| IBIS file stm32mp157xac_tfbga361.ibs
[IBIS ver]   4.2
[File name]   stm32mp157xac_tfbga361.ibs
[File Rev]   2.2
[Date]   07-07-2026
[Source]   Data Created at STMicroelectronics
[Disclaimer]  This information is for modeling purpose only and is
   not guaranted.
   The information is subject to change without notice.
[Copyright]   Copyright 2026 STMicroelectronics Inc.
|   Component stm32mp157xac_tfbga361
[Component] stm32mp157xac_tfbga361
[Manufacturer] STMicroelectronics
[Package]
| variable   typ   min   max
R_pkg  4.84E-01  2.14E-01  8.53E-01
L_pkg  2.71E-09  1.27E-09  5.07E-09
C_pkg  7.70E-13  5.20E-13  3.84E-12
[Pin]   signal_name   model_name
1A2  VDDCORE  power
1A3  VSS  gnd
1A4  VDDCORE  power
1A5  VSS  gnd
1A6  VDDCORE  power
1A7  VSS  gnd
1A8  VDDQ_DDR  power
1B1  VDDCORE  power
1B2  VSS  gnd
1B3  VDDCORE  power
1B4  VSS  gnd
1B5  VDDCORE  power
1B6  VSS  gnd
1B7  VDDQ_DDR  power
1B8  VSS  gnd
1B9  VDDQ_DDR  power
1C1  VSS  gnd
1C2  VDDCORE  power
1C3  VSS  gnd
1C4  VDDCORE  power
1C5  VSS  gnd
1C6  VDDCORE  power
1C7  VSS  gnd
1C8  VDDQ_DDR  power
1C9  VSS  gnd
1D1  VDDCORE  power
1D2  VSS  gnd
1D3  VDDCORE  power
1D4  VSS  gnd
1D5  VDDCORE  power
1D6  VSS  gnd
1D7  VDDCORE  power
1D8  VSS  gnd
1D9  VDDQ_DDR  power
1E1  VSS  gnd
1E2  VDDCORE  power
1E3  VSS  gnd
1E4  VDDCORE  power
1E5  VSS  gnd
1E6  VDDCORE  power
1E7  VSS  gnd
1E8  VDDQ_DDR  power
1E9  VSS  gnd
1F1  VBAT  power
1F2  VSS  gnd
1F3  VDD  power
1F4  VSS  gnd
1F5  VDDCORE  power
1F6  VSS  gnd
1F7  VDDCORE  power
1F8  VSS  gnd
1F9  VDDQ_DDR  power
1G1  VSS_ANA  nc
1G2  VDD_ANA  nc
1G3  VSS  gnd
1G4  VDD  power
1G5  VSS  gnd
1G6  VDDCORE  power
1G7  VSS  gnd
1G8  VDDQ_DDR  power
1G9  VSS  gnd
1H1  VDDA  nc
1H2  VSSA  gnd
1H3  VDD  power
1H4  VSS  gnd
1H5  VDD  power
1H6  VSS  gnd
1H7  VDDCORE  power
1H8  VSS  gnd
1H9  VDDQ_DDR  power
1J2  VDD_OTP  power
1J3  VSS  gnd
1J4  VDD  power
1J5  VSS  gnd
1J6  VDD  power
1J7  VSS  gnd
1J8  VDDQ_DDR  power
A1  VSS  gnd
A2  PH5  io8_ft_i2c
A3  PE13  io8_ft_hslv
A4  PE11  io8_ft
A5  PF1  io8_ft_hslv
A7  PD5  io8_ft_hslv
A8  PA9  io8_ft_hslv
A10  PG6  io8_ft_hslv
A11  PB3  io8_ft_hslv
A13  PA8  io8_ft_hslv
A14  PF2  io8_ft_hslv
A16  DNU  nc
A17  DNU  nc
A19  JTDO-TRACESWO io8_ft_hslv
A20  JTDI  isudqf
A21  DDR_DQ20  PDDRIO_PAD
A22  DDR_DQ23  PDDRIO_PAD
A23  VSS  gnd
AA1  PG14  io8_ft_hslv_et
AA2  PG13  io8_ft_hslv_et
AA3  PH3  io8_ft_hslv
AA4  PA1  io8_ft_hslv
AA5  VSS  gnd
AA6  PC1  io8_ft_hslv
AA7  PB1  io8_ft
AA8  VSS  gnd
AA9  PE9  io8_ft_hslv
AA10  PB13  io8_ft_hslv_et
AA11  PE7  io8_ft_hslv
AA12  VSS  gnd
AA13  PF6  io8_ft_hslv
AA14  PF9  io8_ft_hslv
AA15  VDD3V3_USBHS  power
AA16  VSS_USBHS  gnd
AA17  VDD3V3_USBFS  power
AA18  PA11  io8_i2c_usb_lsfs_bcd_otg20_ft
AA19  PD13  io8_ft_i2c_hslv
AA20  DDR_DQM3  PDDRIO_PAD
AA21  VSS  gnd
AA22  DDR_DQ31  PDDRIO_PAD
AA23  DDR_DQ30  PDDRIO_PAD
AB1  PB11  io8_ft_et_i2c_hslv
AB2  PG4  io8_ft_hslv_et
AB3  PA0  io8_ft_hslv
AB4  PH2  io8_ft_hslv
AB5  PC0  io8_ft_hslv
AB6  PB0  io8_ft
AB7  PC5  io8_ft
AB8  PA7  io8_ft_hslv
AB9  PG8  io8_ft_hslv_et
AB10  PB8  io8_ft_et_i2c_hslv
AB11  PG10  io8_ft_hslv
AB12  PF7  io8_ft_hslv
AB13  BYPASS_REG1V8  isudqf
AB14  VDDA1V8_REG  nc
AB15  VDDA1V1_REG  nc
AB16  USB_DM2  nc
AB17  USB_DM1  nc
AB18  USB_RREF  nc
AB19  PA12  io8_i2c_usb_lsfs_bcd_otg20_ft
AB20  DDR_DQ27  PDDRIO_PAD
AB21  DDR_DQ26  PDDRIO_PAD
AB22  DDR_DQS3P  PDIFF_PAD
AB23  DDR_DQS3N  PDIFF_PAD
AC1  VSS  gnd
AC2  PG0  io8_ft_hslv_et
AC3  PA2  io8_ft_hslv
AC4  PF14  io8_ft_i2c_hslv
AC5  PB12  io8_ft_hslv_et
AC7  PC4  io8_ft
AC8  PA6  io8_ft_hslv
AC10  PD11  io8_ft_hslv
AC11  PF8  io8_ft_hslv
AC13  PE8  io8_ft_hslv
AC14  PG7  io8_ft_hslv
AC16  USB_DP2  nc
AC17  USB_DP1  nc
AC19  OTG_VBUS  io8usb_vbus_otg20_ft
AC20  DDR_VREF  POWER
AC21  DDR_DQ29  PDDRIO_PAD
AC22  DDR_DQ28  PDDRIO_PAD
AC23  VSS  gnd
B1  PH15  io8_ft
B2  PH12  io8_ft_i2c
B3  PH4  io8_ft_i2c
B4  PE12  io8_ft_hslv
B5  PD10  io8_ft_hslv
B6  PD4  io8_ft_hslv
B7  PG15  io8_ft_hslv
B8  PD0  io8_ft_hslv
B9  PD1  io8_ft_hslv
B10  PB9  io8_ft_hslv
B11  PC7  io8_ft_hslv
B12  PB15  io8_ft_hslv
B13  PB4  io8_ft_hslv
B14  PC6  io8_ft_hslv
B15  DNU  nc
B16  DNU  nc
B17  DNU  nc
B18  VDD_Unused  power
B19  NJTRST  isudqf
B20  JTCK-SWCLK  io8_ft
B21  DDR_DQ19  PDDRIO_PAD
B22  DDR_DQ16  PDDRIO_PAD
B23  DDR_DQS2N  PDIFF_PAD
C1  PI0  io8_ft
C2  PH10  io8_ft
C3  PH14  io8_ft
C4  PH11  io8_ft_i2c
C5  PH9  io8_ft
C6  PE14  io8_ft_hslv
C7  VSS  gnd
C8  PE1  io8_ft
C9  PE3  io8_ft_hslv
C10  PE6  io8_ft_hslv
C11  PE5  io8_ft_hslv
C12  VSS  gnd
C13  PB14  io8_ft_hslv
C14  VDDA1V8_Unused  nc
C15  DNU  nc
C16  VSS  gnd
C17  VDD1V2_Unused   nc
C18  VDD1V2_Unused   nc
C19  PA15  io8_ft_hslv
C20  JTMS-SWDIO  io8_ft_hslv
C21  VSS  gnd
C22  DDR_DQS2P  PDIFF_PAD
C23  DDR_DQM2 PDDRIO_PAD
D1  PH13  io8_ft
D2  PD6  io8_ft_hslv
D3  PE15  io8_ft
D4  VSS  gnd
D5  PH8  io8_ft_i2c
D6  PE0  io8_ft_hslv
D7  PF5  io8_ft_hslv
D8  PF0  io8_ft_hslv
D9  PF4  io8_ft_hslv
D10  PD7  io8_ft_hslv
D11  PB7  io8_ft_hslv
D12  PD2  io8_ft_hslv
D13  PC12  io8_ft_hslv
D14  PD3  io8_ft_hslv
D15  PC10  io8_ft_hslv
D16  PC11  io8_ft_hslv
D17  PC9  io8_ft_hslv
D18  PC8  io8_ft_hslv
D19  PE4  io8_ft_hslv
D20  DDR_RESETN  PDDRIO_PAD
D21  DDR_DQ22  PDDRIO_PAD
D22  DDR_DQ17  PDDRIO_PAD
D23  DDR_DQ18  PDDRIO_PAD
E1  PI3  io8_ft_hslv
E2  PI2  io8_ft_hslv
E3  PI1  io8_ft_hslv
E4  PI4  io8_ft
E20  DDR_A7  PDDRIO_PAD
E21  DDR_DQ3  PDDRIO_PAD
E22  DDR_DQ0  PDDRIO_PAD
E23  DDR_DQ21  PDDRIO_PAD
F2  PI7  io8_ft
F3  PI5  io8_ft
F4  PI6  io8_ft
F20  DDR_A13  PDDRIO_PAD
F21  VSS  gnd
F22  DDR_DQ1  PDDRIO_PAD
G1  PZ1  io8_ft_hslv
G2  PZ4  io8_ft_i2c
G3  PZ0  io8_ft_hslv
G4  PZ3  io8_ft_i2c
G20  DDR_A9  PDDRIO_PAD
G21  DDR_DQ7  PDDRIO_PAD
G22  DDR_DQS0P  PDIFF_PAD
G23  DDR_DQS0N  PDIFF_PAD
H1  PZ6  io8_ft_i2c
H2  PZ5  io8_ft_i2c
H3  VSS  gnd
H4  PI9  io8_ft
H20  DDR_A5  PDDRIO_PAD
H21  DDR_DQ2  PDDRIO_PAD
H22  DDR_DQ6  PDDRIO_PAD
H23  DDR_DQM0  PDDRIO_PAD
J2  PD15  io8_ft
J3  PZ7  io8_ft_i2c
J4  PZ2  io8_ft_hslv
J20  DDR_A2  PDDRIO_PAD
J21  DDR_DQ4  PDDRIO_PAD
J22  DDR_DQ5  PDDRIO_PAD
K1  PD9  io8_ft
K2  PC13  io8_ft
K3  PD8  io8_ft
K4  PG12  io8_ft_hslv
K20  DDR_DTO0  PDDRIO_PAD
K21  VSS  gnd
K22  DDR_A3  PDDRIO_PAD
K23  DDR_ZQ  nc
L1  PC15-OSC32_OUT io8_ft
L2  PC14-OSC32_IN  io8_ft
L3  PD14  io8_ft
L4  PI8  io8_ft
L20  DDR_A0  PDDRIO_PAD
L21  DDR_DTO1  PDDRIO_PAD
L22  DDR_ODT  PDDRIO_PAD
L23  DDR_BA0  PDDRIO_PAD
M2  BOOT2  isudqf
|M3  NRST  ioreset_ft_v33
M3  NRST  nc
M4  NRST_CORE  isudqf
M20  DDR_WEN  PDDRIO_PAD
M21  DDR_BA2  PDDRIO_PAD
M22  DDR_CSN  PDDRIO_PAD
N1  BOOT0  isudqf
N2  PA13  io8_ft
N3  PWR_LP  io8_ft
N4  BOOT1  isudqf
N20  DDR_CASN  PDDRIO_PAD
N21  DDR_RASN  PDDRIO_PAD
N22  DDR_CLKP  PDDRIO_PAD
N23  DDR_CLKN  PDDRIO_PAD
P1  PH0-OSC_IN  io8_ft
P2  PH1-OSC_OUT  io8_ft
P3  VSS  gnd
P4  PI11  io8_ft
P20  DDR_A15  PDDRIO_PAD
P21  VSS  gnd
P22  DDR_A1  PDDRIO_PAD
P23  DDR_A12  PDDRIO_PAD
R2  PWR_ON  io8_ft
R3  PDR_ON  isudqf
R4  VREF+  nc
R20  DDR_A11  PDDRIO_PAD
R21  DDR_A14  PDDRIO_PAD
R22  DDR_A10  PDDRIO_PAD
T1  PI10  io8_ft
T2  PA14  io8_ft
T3  PDR_ON_CORE  isudqf
T4  PG3  io8_ft_hslv_et
T20  DDR_CKE  PDDRIO_PAD
T21  DDR_DQ8  PDDRIO_PAD
T22  DDR_DQ10  PDDRIO_PAD
T23  DDR_DQ13  PDDRIO_PAD
U1  PF3  io8_ft_hslv_et
U2  PA3  io8_ft
U3  ANA0  nc
U4  ANA1  nc
U20  DDR_BA1  PDDRIO_PAD
U21  DDR_DQ9  PDDRIO_PAD
U22  DDR_DQS1P  PDIFF_PAD
U23  DDR_DQS1N  PDIFF_PAD
V2  PG2  io8_ft_hslv_et
V3  PA5  io8_ft_hslv
V4  PA4  io8_ft
V20  DDR_A4  PDDRIO_PAD
V21  VSS  gnd
V22  DDR_DQM1 PDDRIO_PAD
W1  PG1  io8_ft_hslv_et
W2  PC3  io8_ft_hslv
W3  VSS  gnd
W4  PH7  io8_ft_hslv
W20  DDR_A6  PDDRIO_PAD
W21  DDR_DQ11  PDDRIO_PAD
W22  DDR_DQ14  PDDRIO_PAD
W23  DDR_DQ12  PDDRIO_PAD
Y1  PE2  io8_ft_et_i2c_hslv
Y2  PC2  io8_ft_hslv_et
Y3  PB10  io8_ft_i2c_hslv
Y4  PF15  io8_ft_hslv
Y5  PF13  io8_ft_hslv
Y6  PG5  io8_ft
Y7  PG11  io8_ft_hslv_et
Y8  PB5  io8_ft_hslv_et
Y9  PF12  io8_ft_hslv
Y10  PF11  io8_ft_hslv
Y11  PH6  io8_ft_hslv
Y12  PF10  io8_ft_hslv
Y13  PG9  io8_ft_hslv
Y14  PB6  io8_ft_i2c_hslv
Y15  PE10  io8_ft_hslv
Y16  PB2  io8_ft_hslv
Y17  PA10  io8usb_id_otg20_ft
Y18  PD12  io8_ft_i2c_hslv
Y19  DDR_ATO  nc
Y20  DDR_A8  PDDRIO_PAD
Y21  DDR_DQ15  PDDRIO_PAD
Y22  DDR_DQ25  PDDRIO_PAD
Y23  DDR_DQ24  PDDRIO_PAD
[Package Model]   500-tfbga-12x12-361-100mhz-181019
[Pin Mapping]   pulldown_ref   pullup_ref   | Comment
1A2  nc  VDDCORE
1A3  VSS  nc
1A4  nc  VDDCORE
1A5  VSS  nc
1A6  nc  VDDCORE
1A7  VSS  nc
1A8  nc  VDDQ_DDR
1B1  nc  VDDCORE
1B2  VSS  nc
1B3  nc  VDDCORE
1B4  VSS  nc
1B5  nc  VDDCORE
1B6  VSS  nc
1B7  nc  VDDQ_DDR
1B8  VSS  nc
1B9  nc  VDDQ_DDR
1C1  VSS  nc
1C2  nc  VDDCORE
1C3  VSS  nc
1C4  nc  VDDCORE
1C5  VSS  nc
1C6  nc  VDDCORE
1C7  VSS  nc
1C8  nc  VDDQ_DDR
1C9  VSS  nc
1D1  nc  VDDCORE
1D2  VSS  nc
1D3  nc  VDDCORE
1D4  VSS  nc
1D5  nc  VDDCORE
1D6  VSS  nc
1D7  nc  VDDCORE
1D8  VSS  nc
1D9  nc  VDDQ_DDR
1E1  VSS  nc
1E2  nc  VDDCORE
1E3  VSS  nc
1E4  nc  VDDCORE
1E5  VSS  nc
1E6  nc  VDDCORE
1E7  VSS  nc
1E8  nc  VDDQ_DDR
1E9  VSS  nc
1F1  nc  VBAT
1F2  VSS  nc
1F3  nc  VDD
1F4  VSS  nc
1F5  nc  VDDCORE
1F6  VSS  nc
1F7  nc  VDDCORE
1F8  VSS  nc
1F9  nc  VDDQ_DDR
1G1  nc  nc
1G2  nc  nc
1G3  VSS  nc
1G4  nc  VDD
1G5  VSS  nc
1G6  nc  VDDCORE
1G7  VSS  nc
1G8  nc  VDDQ_DDR
1G9  VSS  nc
1H1  nc  nc
1H2  VSS  nc
1H3  nc  VDD
1H4  VSS  nc
1H5  nc  VDD
1H6  VSS  nc
1H7  nc  VDDCORE
1H8  VSS  nc
1H9  nc  VDDQ_DDR
1J2  nc  VDD
1J3  VSS  nc
1J4  nc  VDD
1J5  VSS  nc
1J6  nc  VDD
1J7  VSS  nc
1J8  nc  VDDQ_DDR
A1  VSS  nc
A2  VSS  VDD
A3  VSS  VDD
A4  VSS  VDD
A5  VSS  VDD
A7  VSS  VDD
A8  VSS  VDD
A10  VSS  VDD
A11  VSS  VDD
A13  VSS  VDD
A14  VSS  VDD
A16  nc nc
A17   nc nc
A19   nc nc
A20  VSS  VDD
A21  VSS  VDDQ_DDR
A22  VSS  VDDQ_DDR
A23  VSS  nc
AA1  VSS  VDD
AA2  VSS  VDD
AA3  VSS  VDD
AA4  VSS  VDD
AA5  VSS  nc
AA6  VSS  VDD
AA7  VSS  VDD
AA8  VSS  nc
AA9  VSS  VDD
AA10  VSS  VDD
AA11  VSS  VDD
AA12  VSS  nc
AA13  VSS  VDD
AA14  VSS  VDD
AA15  nc  VDD3V3_USBHS
AA16  VSS_USBHS  nc
AA17  nc  VDD3V3_USBFS
AA18  VSS  VDD3V3_USBFS  | Depending on IO usage
| AA18  VSS  VDD  | Depending on IO usage
AA19  VSS  VDD
AA20  VSS  VDDQ_DDR
AA21  VSS  nc
AA22  VSS  VDDQ_DDR
AA23  VSS  VDDQ_DDR
AB1  VSS  VDD
AB2  VSS  VDD
AB3  VSS  VDD
AB4  VSS  VDD
AB5  VSS  VDD
AB6  VSS  VDD
AB7  VSS  VDD
AB8  VSS  VDD
AB9  VSS  VDD
AB10 VSS  VDD
AB11 VSS  VDD
AB12 VSS  VDD
AB13 VSS  VDD
AB14 nc nc
AB15 nc nc
AB16 nc nc
AB17 nc nc
AB18 nc nc
AB19  VSS  VDD3V3_USBFS  | Depending on IO usage
| AB19  VSS  VDD  | Depending on IO usage
AB20  VSS  VDDQ_DDR
AB21  VSS  VDDQ_DDR
AB22  VSS  VDDQ_DDR
AB23  VSS  VDDQ_DDR
AC1  VSS  nc
AC2  VSS  VDD
AC3  VSS  VDD
AC4  VSS  VDD
AC5  VSS  VDD
AC7  VSS  VDD
AC8  VSS  VDD
AC10  VSS  VDD
AC11  VSS  VDD
AC13  VSS  VDD
AC14  VSS  VDD
AC16 nc nc
AC17 nc nc
AC19   nc nc
AC20 nc VDDQ_DDR
AC21  VSS  VDDQ_DDR
AC22  VSS  VDDQ_DDR
AC23  VSS  nc
B1  VSS  VDD
B2  VSS  VDD
B3  VSS  VDD
B4  VSS  VDD
B5  VSS  VDD
B6  VSS  VDD
B7  VSS  VDD
B8  VSS  VDD
B9  VSS  VDD
B10  VSS  VDD
B11  VSS  VDD
B12  VSS  VDD
B13  VSS  VDD
B14  VSS  VDD
B15   nc nc
B16   nc nc
B17   nc nc
B18  nc  VDD_Unused
B19  VSS  VDD
B20   nc nc
B21  VSS  VDDQ_DDR
B22  VSS  VDDQ_DDR
B23  VSS  VDDQ_DDR
C1  VSS  VDD
C2  VSS  VDD
C3  VSS  VDD
C4  VSS  VDD
C5  VSS  VDD
C6  VSS  VDD
C7  VSS  nc
C8  VSS  VDD
C9  VSS  VDD
C10  VSS  VDD
C11  VSS  VDD
C12  VSS  nc
C13  VSS  VDD
C14  nc  nc
C15  nc nc
C16  VSS  nc
C17  nc  nc
C18  nc  nc
C19  VSS  VDD
C20   nc nc
C21  VSS  nc
C22  VSS  VDDQ_DDR
C23   VSS  VDDQ_DDR
D1  VSS  VDD
D2  VSS  VDD
D3  VSS  VDD
D4  VSS  nc
D5  VSS  VDD
D6  VSS  VDD
D7  VSS  VDD
D8  VSS  VDD
D9  VSS  VDD
D10  VSS  VDD
D11  VSS  VDD
D12  VSS  VDD
D13  VSS  VDD
D14  VSS  VDD
D15  VSS  VDD
D16  VSS  VDD
D17  VSS  VDD
D18  VSS  VDD
D19  VSS  VDD
D20  VSS  VDDQ_DDR
D21  VSS  VDDQ_DDR
D22  VSS  VDDQ_DDR
D23  VSS  VDDQ_DDR
E1  VSS  VDD
E2  VSS  VDD
E3  VSS  VDD
E4  VSS  VDD
E20  VSS  VDDQ_DDR
E21  VSS  VDDQ_DDR
E22  VSS  VDDQ_DDR
E23  VSS  VDDQ_DDR
F2  VSS  VDD
F3  VSS  VDD
F4  VSS  VDD
F20  VSS  VDDQ_DDR
F21  VSS  nc
F22  VSS  VDDQ_DDR
G1  VSS  VDD
G2  VSS  VDD
G3  VSS  VDD
G4  VSS  VDD
G20  VSS  VDDQ_DDR
G21  VSS  VDDQ_DDR
G22  VSS  VDDQ_DDR
G23  VSS  VDDQ_DDR
H1  VSS  VDD
H2  VSS  VDD
H3  VSS  nc
H4  VSS  VDD
H20  VSS  VDDQ_DDR
H21  VSS  VDDQ_DDR
H22  VSS  VDDQ_DDR
H23  VSS  VDDQ_DDR
J2  VSS  VDD
J3  VSS  VDD
J4  VSS  VDD
J20  VSS  VDDQ_DDR
J21  VSS  VDDQ_DDR
J22  VSS  VDDQ_DDR
K1  VSS  VDD
K2  nc  nc
K3  VSS  VDD
K4  VSS  VDD
K20  VSS  VDDQ_DDR
K21  VSS  nc
K22  VSS  VDDQ_DDR
K23  nc  nc
L1   nc nc
L2   nc nc
L3  VSS  VDD
L4  nc  nc
L20  VSS  VDDQ_DDR
L21  VSS  VDDQ_DDR
L22  VSS  VDDQ_DDR
L23  VSS  VDDQ_DDR
M2  VSS  VDD
M3  nc  nc
M4  VSS  VDD
M20  VSS  VDDQ_DDR
M21  VSS  VDDQ_DDR
M22  VSS  VDDQ_DDR
N1  VSS  VDD
N2  VSS  VDD
N3  VSS  VDD
N4  VSS  VDD
N20  VSS  VDDQ_DDR
N21  VSS  VDDQ_DDR
N22  VSS  VDDQ_DDR
N23  VSS  VDDQ_DDR
P1   nc nc
P2   nc nc
P3  VSS  nc
P4  VSS  VDD
P20  VSS  VDDQ_DDR
P21  VSS  nc
P22  VSS  VDDQ_DDR
P23  VSS  VDDQ_DDR
R2  VSS  VDD
R3  VSS  VDD
R4   nc nc
R20  VSS  VDDQ_DDR
R21  VSS  VDDQ_DDR
R22  VSS  VDDQ_DDR
T1  VSS  VDD
T2  VSS  VDD
T3  VSS  VDD
T4  VSS  VDD
T20  VSS  VDDQ_DDR
T21  VSS  VDDQ_DDR
T22  VSS  VDDQ_DDR
T23  VSS  VDDQ_DDR
U1  VSS  VDD
U2  VSS  VDD
U3 nc nc
U4 nc nc
U20  VSS  VDDQ_DDR
U21  VSS  VDDQ_DDR
U22  VSS  VDDQ_DDR
U23  VSS  VDDQ_DDR
V2  VSS  VDD
V3  VSS  VDD
V4  VSS  VDD
V20  VSS  VDDQ_DDR
V21  VSS  nc
V22 VSS  VDDQ_DDR
W1  VSS  VDD
W2  VSS  VDD
W3  VSS  nc
W4  VSS  VDD
W20  VSS  VDDQ_DDR
W21  VSS  VDDQ_DDR
W22  VSS  VDDQ_DDR
W23  VSS  VDDQ_DDR
Y1  VSS  VDD
Y2  VSS  VDD
Y3  VSS  VDD
Y4  VSS  VDD
Y5  VSS  VDD
Y6  VSS  VDD
Y7  VSS  VDD
Y8  VSS  VDD
Y9  VSS  VDD
Y10  VSS  VDD
Y11  VSS  VDD
Y12  VSS  VDD
Y13  VSS  VDD
Y14  VSS  VDD
Y15  VSS  VDD
Y16  VSS  VDD
Y17  VSS  VDD3V3_USBFS  | Depending on IO usage
| Y17  VSS  VDD  | Depending on IO usage
Y18  VSS  VDD
Y19  nc nc
Y20  VSS  VDDQ_DDR
Y21  VSS  VDDQ_DDR
Y22  VSS  VDDQ_DDR
Y23  VSS  VDDQ_DDR
[Diff_pin]   inv_pin   vdiff   tdelay_typ   tdelay_min   tdelay_max
N22   N23   0.320V   0ns   NA   NA  |CLK
G22   G23   0.320V   0ns   NA   NA  |DQS0
U22   U23   0.320V   0ns   NA   NA  |DQS1
C22   B23   0.320V   0ns   NA   NA  |DQS2
AB22   AB23   0.320V   0ns   NA   NA  |DQS3
[Model Selector] io8usb_id_otg20_ft
io8_ft_ls_1v2   "GPIO - 5V tolerant - 1.2V range - Low speed"
io8_ft_ms_1v2   "GPIO - 5V tolerant - 1.2V range - Med speed"
io8_ft_hs_1v2   "GPIO - 5V tolerant - 1.2V range - High speed"
io8_ft_fs_1v2   "GPIO - 5V tolerant - 1.2V range - Fast speed"
io8_ft_hs_1v8   "GPIO - 5V tolerant - 1.8V range - High speed"
io8_ft_fs_1v8   "GPIO - 5V tolerant - 1.8V range - Fast speed"
io8_ft_ms_1v8   "GPIO - 5V tolerant - 1.8V range - Med speed"
io8_ft_ls_1v8   "GPIO - 5V tolerant - 1.8V range - Low speed"
io8_ft_hs_3v3   "GPIO - 5V tolerant - 3.3V range - High speed"
io8_ft_fs_3v3   "GPIO - 5V tolerant - 3.3V range - Fast speed"
io8_ft_ms_3v3   "GPIO - 5V tolerant - 3.3V range - Med speed"
io8_ft_ls_3v3   "GPIO - 5V tolerant - 3.3V range - Low speed"
[Model Selector] io8usb_vbus_otg20_ft
io8_ft_ls_1v2   "GPIO - 5V tolerant - 1.2V range - Low speed"
io8_ft_ms_1v2   "GPIO - 5V tolerant - 1.2V range - Med speed"
io8_ft_hs_1v2   "GPIO - 5V tolerant - 1.2V range - High speed"
io8_ft_fs_1v2   "GPIO - 5V tolerant - 1.2V range - Fast speed"
io8_ft_hs_1v8   "GPIO - 5V tolerant - 1.8V range - High speed"
io8_ft_fs_1v8   "GPIO - 5V tolerant - 1.8V range - Fast speed"
io8_ft_ms_1v8   "GPIO - 5V tolerant - 1.8V range - Med speed"
io8_ft_ls_1v8   "GPIO - 5V tolerant - 1.8V range - Low speed"
io8_ft_hs_3v3   "GPIO - 5V tolerant - 3.3V range - High speed"
io8_ft_fs_3v3   "GPIO - 5V tolerant - 3.3V range - Fast speed"
io8_ft_ms_3v3   "GPIO - 5V tolerant - 3.3V range - Med speed"
io8_ft_ls_3v3   "GPIO - 5V tolerant - 3.3V range - Low speed"
[Model Selector] io8_ft
io8_ft_ls_1v2   "GPIO - 5V tolerant - 1.2V range - Low speed"
io8_ft_ms_1v2   "GPIO - 5V tolerant - 1.2V range - Med speed"
io8_ft_hs_1v2   "GPIO - 5V tolerant - 1.2V range - High speed"
io8_ft_fs_1v2   "GPIO - 5V tolerant - 1.2V range - Fast speed"
io8_ft_hs_1v8   "GPIO - 5V tolerant - 1.8V range - High speed"
io8_ft_fs_1v8   "GPIO - 5V tolerant - 1.8V range - Fast speed"
io8_ft_ms_1v8   "GPIO - 5V tolerant - 1.8V range - Med speed"
io8_ft_ls_1v8   "GPIO - 5V tolerant - 1.8V range - Low speed"
io8_ft_hs_3v3   "GPIO - 5V tolerant - 3.3V range - High speed"
io8_ft_fs_3v3   "GPIO - 5V tolerant - 3.3V range - Fast speed"
io8_ft_ms_3v3   "GPIO - 5V tolerant - 3.3V range - Med speed"
io8_ft_ls_3v3   "GPIO - 5V tolerant - 3.3V range - Low speed"
[Model Selector] io8_ft_hslv
io8_ft_ls_1v2   "GPIO - 5V tolerant - 1.2V range - Low speed"
io8_ft_ms_1v2   "GPIO - 5V tolerant - 1.2V range - Med speed"
io8_ft_hs_1v2   "GPIO - 5V tolerant - 1.2V range - High speed"
io8_ft_fs_1v2   "GPIO - 5V tolerant - 1.2V range - Fast speed"
io8_ft_hs_1v8   "GPIO - 5V tolerant - 1.8V range - High speed"
io8_ft_fs_1v8   "GPIO - 5V tolerant - 1.8V range - Fast speed"
io8_ft_ms_1v8   "GPIO - 5V tolerant - 1.8V range - Med speed"
io8_ft_ls_1v8   "GPIO - 5V tolerant - 1.8V range - Low speed"
io8_ft_hs_3v3   "GPIO - 5V tolerant - 3.3V range - High speed"
io8_ft_fs_3v3   "GPIO - 5V tolerant - 3.3V range - Fast speed"
io8_ft_ms_3v3   "GPIO - 5V tolerant - 3.3V range - Med speed"
io8_ft_ls_3v3   "GPIO - 5V tolerant - 3.3V range - Low speed"
io8_ft_hslv_hs_1v2   "GPIO - hslv opt - 5V tolerant - 1.2V range - High speed"
io8_ft_hslv_fs_1v2   "GPIO - hslv opt - 5V tolerant - 1.2V range - Fast speed"
io8_ft_hslv_ms_1v2   "GPIO - hslv opt - 5V tolerant - 1.2V range - Med speed"
io8_ft_hslv_ls_1v2   "GPIO - hslv opt - 5V tolerant - 1.2V range - Low speed"
io8_ft_hslv_hs_1v8   "GPIO - hslv opt - 5V tolerant - 1.8V range - High speed"
io8_ft_hslv_fs_1v8   "GPIO - hslv opt - 5V tolerant - 1.8V range - Fast speed"
io8_ft_hslv_ms_1v8   "GPIO - hslv opt - 5V tolerant - 1.8V range - Med speed"
io8_ft_hslv_ls_1v8   "GPIO - hslv opt - 5V tolerant - 1.8V range - Low speed"
io8_ft_hslv_hs_2v5   "GPIO - hslv opt - 5V tolerant - 2.5V range - High speed"
io8_ft_hslv_fs_2v5   "GPIO - hslv opt - 5V tolerant - 2.5V range - Fast speed"
io8_ft_hslv_ms_2v5   "GPIO - hslv opt - 5V tolerant - 2.5V range - Med speed"
io8_ft_hslv_ls_2v5   "GPIO - hslv opt - 5V tolerant - 2.5V range - Low speed"
[Model Selector] io8_ft_hslv_et
io8_ft_et_ls_1v2   "GPIO - Ethernet - 5V tol - 1.2V range - Low speed"
io8_ft_et_ms_1v2   "GPIO - Ethernet - 5V tol - 1.2V range - Med speed"
io8_ft_et_hs_1v2   "GPIO - Ethernet - 5V tol - 1.2V range - High speed"
io8_ft_et_fs_1v2   "GPIO - Ethernet - 5V tol - 1.2V range - Fast speed"
io8_ft_et_hs_1v8   "GPIO - Ethernet - 5V tol - 1.8V range - High speed"
io8_ft_et_fs_1v8   "GPIO - Ethernet - 5V tol - 1.8V range - Fast speed"
io8_ft_et_ms_1v8   "GPIO - Ethernet - 5V tol - 1.8V range - Med speed"
io8_ft_et_ls_1v8   "GPIO - Ethernet - 5V tol - 1.8V range - Low speed"
io8_ft_et_hs_3v3   "GPIO - Ethernet - 5V tol - 3.3V range - High speed"
io8_ft_et_fs_3v3   "GPIO - Ethernet - 5V tol - 3.3V range - Fast speed"
io8_ft_et_ms_3v3   "GPIO - Ethernet - 5V tol - 3.3V range - Med speed"
io8_ft_et_ls_3v3   "GPIO - Ethernet - 5V tol - 3.3V range - Low speed"
io8_ft_et_hslv_ls_1v2   "GPIO - hslv opt - Ethernet - 5V tol - 1.2V range - Low speed"
io8_ft_et_hslv_hs_1v2   "GPIO - hslv opt - Ethernet - 5V tol - 1.2V range - High speed"
io8_ft_et_hslv_fs_1v2   "GPIO - hslv opt - Ethernet - 5V tol - 1.2V range - Fast speed"
io8_ft_et_hslv_ms_1v2   "GPIO - hslv opt - Ethernet - 5V tol - 1.2V range - Med speed"
io8_ft_et_hslv_ls_1v8   "GPIO - hslv opt - Ethernet - 5V tol - 1.8V range - Low speed"
io8_ft_et_hslv_hs_1v8   "GPIO - hslv opt - Ethernet - 5V tol - 1.8V range - High speed"
io8_ft_et_hslv_fs_1v8   "GPIO - hslv opt - Ethernet - 5V tol - 1.2V range - Fast speed"
io8_ft_et_hslv_ms_1v8   "GPIO - hslv opt - Ethernet - 5V tol - 1.8V range - Med speed"
io8_ft_et_hslv_hs_2v5   "GPIO - hslv opt - Ethernet - 5V tol - 2.5V range - High speed"
io8_ft_et_hslv_fs_2v5   "GPIO - hslv opt - Ethernet - 5V tol - 2.5V range - Fast speed"
io8_ft_et_hslv_ms_2v5   "GPIO - hslv opt - Ethernet - 5V tol - 2.5V range - Med speed"
io8_ft_et_hslv_ls_2v5   "GPIO - hslv opt - Ethernet - 5V tol - 2.5V range - Low speed"
[Model Selector] io8_ft_et_i2c_hslv
io8_ft_et_ls_1v2   "GPIO - 5V tol - 1.2V range - Low speed"
io8_ft_et_ms_1v2   "GPIO - 5V tol - 1.2V range - Med speed"
io8_ft_et_hs_1v2   "GPIO - 5V tol - 1.2V range - High speed"
io8_ft_et_fs_1v2   "GPIO - 5V tol - 1.2V range - Fast speed"
io8_ft_et_hs_1v8   "GPIO - 5V tol - 1.8V range - High speed"
io8_ft_et_fs_1v8   "GPIO - 5V tol - 1.8V range - Fast speed"
io8_ft_et_ms_1v8   "GPIO - 5V tol - 1.8V range - Med speed"
io8_ft_et_ls_1v8   "GPIO - 5V tol - 1.8V range - Low speed"
io8_ft_et_hs_3v3   "GPIO - 5V tol - 3.3V range - High speed"
io8_ft_et_fs_3v3   "GPIO - 5V tol - 3.3V range - Fast speed"
io8_ft_et_ms_3v3   "GPIO - 5V tol - 3.3V range - Med speed"
io8_ft_et_ls_3v3   "GPIO - 5V tol - 3.3V range - Low speed"
io8_ft_et_hslv_ls_1v2   "GPIO - hslv opt -Ethernet - 5V tol - 1.2V range - Low speed"
io8_ft_et_hslv_hs_1v2   "GPIO - hslv opt -Ethernet - 5V tol - 1.2V range - High speed"
io8_ft_et_hslv_fs_1v2   "GPIO - hslv opt -Ethernet - 5V tol - 1.2V range - Fast speed"
io8_ft_et_hslv_ms_1v2   "GPIO - hslv opt -Ethernet - 5V tol - 1.2V range - Med speed"
io8_ft_et_hslv_ls_1v8   "GPIO - hslv opt -Ethernet - 5V tol - 1.8V range - Low speed"
io8_ft_et_hslv_hs_1v8   "GPIO - hslv opt -Ethernet - 5V tol - 1.8V range - High speed"
io8_ft_et_hslv_fs_1v8   "GPIO - hslv opt -Ethernet - 5V tol - 1.2V range - Fast speed"
io8_ft_et_hslv_ms_1v8   "GPIO - hslv opt -Ethernet - 5V tol - 1.8V range - Med speed"
io8_ft_et_hslv_hs_2v5   "GPIO - hslv opt -Ethernet - 5V tol - 2.5V range - High speed"
io8_ft_et_hslv_fs_2v5   "GPIO - hslv opt  -Ethernet- 5V tol - 2.5V range - Fast speed"
io8_ft_et_hslv_ms_2v5   "GPIO - hslv opt -Ethernet - 5V tol - 2.5V range - Med speed"
io8_ft_et_hslv_ls_2v5   "GPIO - hslv opt -Ethernet - 5V tol - 2.5V range - Low speed"
io8_ft_i2c_1v2   "GPIO - 5V tolerant - 1.2V range - Open drain"
io8_ft_i2c_1v8   "GPIO - 5V tolerant - 1.8V range - Open drain"
io8_ft_i2c_3v3   "GPIO - 5V tolerant - 3.3V range - Open drain"
io8_ft_i2c_hslv_1v2   "GPIO - hslv opt - 5V tolerant - 1.2V range - Open drain"
io8_ft_i2c_hslv_1v8   "GPIO - hslv opt - 5V tolerant - 1.8V range - Open drain"
io8_ft_i2c_hslv_2v5   "GPIO - hslv opt - 5V tolerant - 2.5V range - Open drain"
[Model Selector] io8_ft_i2c
io8_ft_ls_1v2   "GPIO - 5V tolerant - 1.2V range - Low speed"
io8_ft_ms_1v2   "GPIO - 5V tolerant - 1.2V range - Med speed"
io8_ft_hs_1v2   "GPIO - 5V tolerant - 1.2V range - High speed"
io8_ft_fs_1v2   "GPIO - 5V tolerant - 1.2V range - Fast speed"
io8_ft_hs_1v8   "GPIO - 5V tolerant - 1.8V range - High speed"
io8_ft_fs_1v8   "GPIO - 5V tolerant - 1.8V range - Fast speed"
io8_ft_ms_1v8   "GPIO - 5V tolerant - 1.8V range - Med speed"
io8_ft_ls_1v8   "GPIO - 5V tolerant - 1.8V range - Low speed"
io8_ft_hs_3v3   "GPIO - 5V tolerant - 3.3V range - High speed"
io8_ft_fs_3v3   "GPIO - 5V tolerant - 3.3V range - Fast speed"
io8_ft_ms_3v3   "GPIO - 5V tolerant - 3.3V range - Med speed"
io8_ft_ls_3v3   "GPIO - 5V tolerant - 3.3V range - Low speed"
io8_ft_i2c_1v2   "GPIO - 5V tolerant - 1.2V range - Open drain"
io8_ft_i2c_1v8   "GPIO - 5V tolerant - 1.8V range - Open drain"
io8_ft_i2c_3v3   "GPIO - 5V tolerant - 3.3V range - Open drain"
[Model Selector] io8_ft_i2c_hslv
io8_ft_ls_1v2   "GPIO - 5V tolerant - 1.2V range - Low speed"
io8_ft_ms_1v2   "GPIO - 5V tolerant - 1.2V range - Med speed"
io8_ft_hs_1v2   "GPIO - 5V tolerant - 1.2V range - High speed"
io8_ft_fs_1v2   "GPIO - 5V tolerant - 1.2V range - Fast speed"
io8_ft_hs_1v8   "GPIO - 5V tolerant - 1.8V range - High speed"
io8_ft_fs_1v8   "GPIO - 5V tolerant - 1.8V range - Fast speed"
io8_ft_ms_1v8   "GPIO - 5V tolerant - 1.8V range - Med speed"
io8_ft_ls_1v8   "GPIO - 5V tolerant - 1.8V range - Low speed"
io8_ft_hs_3v3   "GPIO - 5V tolerant - 3.3V range - High speed"
io8_ft_fs_3v3   "GPIO - 5V tolerant - 3.3V range - Fast speed"
io8_ft_ms_3v3   "GPIO - 5V tolerant - 3.3V range - Med speed"
io8_ft_ls_3v3   "GPIO - 5V tolerant - 3.3V range - Low speed"
io8_ft_hslv_hs_1v2   "GPIO - hslv opt - 5V tolerant - 1.2V range - High speed"
io8_ft_hslv_fs_1v2   "GPIO - hslv opt - 5V tolerant - 1.2V range - Fast speed"
io8_ft_hslv_ms_1v2   "GPIO - hslv opt - 5V tolerant - 1.2V range - Med speed"
io8_ft_hslv_ls_1v2   "GPIO - hslv opt - 5V tolerant - 1.2V range - Low speed"
io8_ft_hslv_hs_1v8   "GPIO - hslv opt - 5V tolerant - 1.8V range - High speed"
io8_ft_hslv_fs_1v8   "GPIO - hslv opt - 5V tolerant - 1.8V range - Fast speed"
io8_ft_hslv_ms_1v8   "GPIO - hslv opt - 5V tolerant - 1.8V range - Med speed"
io8_ft_hslv_ls_1v8   "GPIO - hslv opt - 5V tolerant - 1.8V range - Low speed"
io8_ft_hslv_hs_2v5   "GPIO - hslv opt - 5V tolerant - 2.5V range - High speed"
io8_ft_hslv_fs_2v5   "GPIO - hslv opt - 5V tolerant - 2.5V range - Fast speed"
io8_ft_hslv_ms_2v5   "GPIO - hslv opt - 5V tolerant - 2.5V range - Med speed"
io8_ft_hslv_ls_2v5   "GPIO - hslv opt - 5V tolerant - 2.5V range - Low speed"
io8_ft_i2c_1v2   "GPIO - 5V tolerant - 1.2V range - Open drain"
io8_ft_i2c_1v8   "GPIO - 5V tolerant - 1.8V range - Open drain"
io8_ft_i2c_3v3   "GPIO - 5V tolerant - 3.3V range - Open drain"
io8_ft_i2c_hslv_1v2   "GPIO - hslv opt - 5V tolerant - 1.2V range - Open drain"
io8_ft_i2c_hslv_1v8   "GPIO - hslv opt - 5V tolerant - 1.8V range - Open drain"
io8_ft_i2c_hslv_2v5   "GPIO - hslv opt - 5V tolerant - 2.5V range - Open drain"
[Model Selector] io8_i2c_usb_lsfs_bcd_otg20_ft
io8_ft_ls_1v2   "GPIO - 5V tolerant - 1.2V range - Low speed"
io8_ft_ms_1v2   "GPIO - 5V tolerant - 1.2V range - Med speed"
io8_ft_hs_1v2   "GPIO - 5V tolerant - 1.2V range - High speed"
io8_ft_fs_1v2   "GPIO - 5V tolerant - 1.2V range - Fast speed"
io8_ft_hs_1v8   "GPIO - 5V tolerant - 1.8V range - High speed"
io8_ft_fs_1v8   "GPIO - 5V tolerant - 1.8V range - Fast speed"
io8_ft_ms_1v8   "GPIO - 5V tolerant - 1.8V range - Med speed"
io8_ft_ls_1v8   "GPIO - 5V tolerant - 1.8V range - Low speed"
io8_ft_hs_3v3   "GPIO - 5V tolerant - 3.3V range - High speed"
io8_ft_fs_3v3   "GPIO - 5V tolerant - 3.3V range - Fast speed"
io8_ft_ms_3v3   "GPIO - 5V tolerant - 3.3V range - Med speed"
io8_ft_ls_3v3   "GPIO - 5V tolerant - 3.3V range - Low speed"
io8_ft_i2c_1v2   "GPIO - 5V tolerant - 1.2V range - Open drain"
io8_ft_i2c_1v8   "GPIO - 5V tolerant - 1.8V range - Open drain"
io8_ft_i2c_3v3   "GPIO - 5V tolerant - 3.3V range - Open drain"
io8usb_ft_hs_3v3   "USB full speed"
io8usb_ft_ls_3v3   "USB low speed"
|[Model Selector] ioreset_ft_v33
|ioreset_ft_v33_1v2   "Reset PAD. 5V tolerant. 1.2V range"
|ioreset_ft_v33_1v8   "Reset PAD. 5V tolerant. 1.8V range"
|ioreset_ft_v33_3v3   "Reset PAD. 5V tolerant. 3.3V range"
[Model Selector] isudqf
isudqf_ft_1v2   "Input Buffer - 5V tolerant - 1.2V range"
isudqf_ft_1v8   "Input Buffer - 5V tolerant - 1.8V range"
isudqf_ft_3v3   "Input Buffer - 5V tolerant - 3.3V range"
[Model Selector] PDIFF_PAD
MSD_D3RF2_18   DDR2 MSD_D3R_PDIFF Z0=18-Ohm
MSD_D3RF2_40   DDR2 MSD_D3R_PDIFF Z0=40-Ohm
MSD_D3RF2_48   DDR2 MSD_D3R_PDIFF Z0=48-Ohm
MSD_D3RF2_ODT150   DDR2 MSD_D3R_PDIFF cell 150-Ohm ODT Receiver
MSD_D3RF2_ODT50   DDR2 MSD_D3R_PDIFF cell 50-Ohm ODT Receiver
MSD_D3RF2_ODT75   DDR2 MSD_D3R_PDIFF cell 75-Ohm ODT Receiver
MSD_D3RF2_ODTOFF   DDR2 MSD_D3R_PDIFF cell ODT off Receiver
MSD_D3RF3_34   DDR3 MSD_D3R_PDIFF cell  Z0=34-Ohm
MSD_D3RF3_40   DDR3 MSD_D3R_PDIFF cell  Z0=40-Ohm
MSD_D3RF3_48   DDR3 MSD_D3R_PDIFF cell  Z0=48-Ohm
MSD_D3RF3L_34   DDR3L MSD_D3R_PDIFF cell  Z0=34-Ohm
MSD_D3RF3L_40   DDR3L MSD_D3R_PDIFF cell  Z0=40-Ohm
MSD_D3RF3L_48   DDR3L MSD_D3R_PDIFF cell  Z0=48-Ohm
MSD_D3RF3L_ODT120   DDR3L MSD_D3R_PDIFF cell 120-Ohm ODT Receiver
MSD_D3RF3L_ODT40   DDR3L MSD_D3R_PDIFF cell 40-Ohm ODT Receiver
MSD_D3RF3L_ODT60   DDR3L MSD_D3R_PDIFF cell 60-Ohm ODT Receiver
MSD_D3RF3L_ODTOFF   DDR3L MSD_D3R_PDIFF cell ODT off Receiver
MSD_D3RF3_ODT120   DDR3 MSD_D3R_PDIFF cell 120-Ohm ODT Receiver
MSD_D3RF3_ODT40   DDR3 MSD_D3R_PDIFF cell 40-Ohm ODT Receiver
MSD_D3RF3_ODT60   DDR3 MSD_D3R_PDIFF cell 60-Ohm ODT Receiver
MSD_D3RF3_ODTOFF   DDR3 MSD_D3R_PDIFF cell ODT off Receiver
MSD_D3RFL2_34   LPDDR2 MSD_D3R_PDIFF cell  Z0=34-Ohm
MSD_D3RFL2_40   LPDDR2 MSD_D3R_PDIFF cell  Z0=40-Ohm
MSD_D3RFL2_48   LPDDR2 MSD_D3R_PDIFF cell  Z0=48-Ohm
MSD_D3RFL2_60   LPDDR2 MSD_D3R_PDIFF cell  Z0=60-Ohm
MSD_D3RFL2_80   LPDDR2 MSD_D3R_PDIFF cell  Z0=80-Ohm
MSD_D3RFL2_ODTOFF   LPDDR2 MSD_D3R_PDIFF cell ODT off Receiver
MSD_D3RFL_48   LPDDR MSD_D3R_PDIFF cell  Z0=48-Ohm
MSD_D3RFL_ODTOFF   LPDDR MSD_D3R_PDIFF cell ODT off Receiver
MSD_D3RF2_18_OPEN   DDR2 MSD_D3R_PDIFF_PDQSR Z0=18-Ohm
MSD_D3RF2_40_OPEN   DDR2 MSD_D3R_PDIFF_PDQSR Z0=40-Ohm
MSD_D3RF2_48_OPEN   DDR2 MSD_D3R_PDIFF_PDQSR Z0=48-Ohm
MSD_D3RF2_18_PD344   DDR2 MSD_D3R_PDIFF_PDQSR Z0=18-Ohm
MSD_D3RF2_40_PD344   DDR2 MSD_D3R_PDIFF_PDQSR Z0=40-Ohm
MSD_D3RF2_48_PD344   DDR2 MSD_D3R_PDIFF_PDQSR Z0=48-Ohm
MSD_D3RF2_18_PD393   DDR2 MSD_D3R_PDIFF_PDQSR Z0=18-Ohm
MSD_D3RF2_40_PD393   DDR2 MSD_D3R_PDIFF_PDQSR Z0=40-Ohm
MSD_D3RF2_48_PD393   DDR2 MSD_D3R_PDIFF_PDQSR Z0=48-Ohm
MSD_D3RF2_18_PD458   DDR2 MSD_D3R_PDIFF_PDQSR Z0=18-Ohm
MSD_D3RF2_40_PD458   DDR2 MSD_D3R_PDIFF_PDQSR Z0=40-Ohm
MSD_D3RF2_48_PD458   DDR2 MSD_D3R_PDIFF_PDQSR Z0=48-Ohm
MSD_D3RF2_18_PD500   DDR2 MSD_D3R_PDIFF_PDQSR Z0=18-Ohm
MSD_D3RF2_40_PD500   DDR2 MSD_D3R_PDIFF_PDQSR Z0=40-Ohm
MSD_D3RF2_48_PD500   DDR2 MSD_D3R_PDIFF_PDQSR Z0=48-Ohm
MSD_D3RF2_18_PD550   DDR2 MSD_D3R_PDIFF_PDQSR Z0=18-Ohm
MSD_D3RF2_40_PD550   DDR2 MSD_D3R_PDIFF_PDQSR Z0=40-Ohm
MSD_D3RF2_48_PD550   DDR2 MSD_D3R_PDIFF_PDQSR Z0=48-Ohm
MSD_D3RF2_18_PD611   DDR2 MSD_D3R_PDIFF_PDQSR Z0=18-Ohm
MSD_D3RF2_40_PD611   DDR2 MSD_D3R_PDIFF_PDQSR Z0=40-Ohm
MSD_D3RF2_48_PD611   DDR2 MSD_D3R_PDIFF_PDQSR Z0=48-Ohm
MSD_D3RF2_18_PD688   DDR2 MSD_D3R_PDIFF_PDQSR Z0=18-Ohm
MSD_D3RF2_40_PD688   DDR2 MSD_D3R_PDIFF_PDQSR Z0=40-Ohm
MSD_D3RF2_48_PD688   DDR2 MSD_D3R_PDIFF_PDQSR Z0=48-Ohm
MSD_D3RF2_18_PU344   DDR2 MSD_D3R_PDIFF_PDQSR Z0=18-Ohm
MSD_D3RF2_40_PU344   DDR2 MSD_D3R_PDIFF_PDQSR Z0=40-Ohm
MSD_D3RF2_48_PU344   DDR2 MSD_D3R_PDIFF_PDQSR Z0=48-Ohm
MSD_D3RF2_18_PU393   DDR2 MSD_D3R_PDIFF_PDQSR Z0=18-Ohm
MSD_D3RF2_40_PU393   DDR2 MSD_D3R_PDIFF_PDQSR Z0=40-Ohm
MSD_D3RF2_48_PU393   DDR2 MSD_D3R_PDIFF_PDQSR Z0=48-Ohm
MSD_D3RF2_18_PU458   DDR2 MSD_D3R_PDIFF_PDQSR Z0=18-Ohm
MSD_D3RF2_40_PU458   DDR2 MSD_D3R_PDIFF_PDQSR Z0=40-Ohm
MSD_D3RF2_48_PU458   DDR2 MSD_D3R_PDIFF_PDQSR Z0=48-Ohm
MSD_D3RF2_18_PU500   DDR2 MSD_D3R_PDIFF_PDQSR Z0=18-Ohm
MSD_D3RF2_40_PU500   DDR2 MSD_D3R_PDIFF_PDQSR Z0=40-Ohm
MSD_D3RF2_48_PU500   DDR2 MSD_D3R_PDIFF_PDQSR Z0=48-Ohm
MSD_D3RF2_18_PU550   DDR2 MSD_D3R_PDIFF_PDQSR Z0=18-Ohm
MSD_D3RF2_40_PU550   DDR2 MSD_D3R_PDIFF_PDQSR Z0=40-Ohm
MSD_D3RF2_48_PU550   DDR2 MSD_D3R_PDIFF_PDQSR Z0=48-Ohm
MSD_D3RF2_18_PU611   DDR2 MSD_D3R_PDIFF_PDQSR Z0=18-Ohm
MSD_D3RF2_40_PU611   DDR2 MSD_D3R_PDIFF_PDQSR Z0=40-Ohm
MSD_D3RF2_48_PU611   DDR2 MSD_D3R_PDIFF_PDQSR Z0=48-Ohm
MSD_D3RF2_18_PU688   DDR2 MSD_D3R_PDIFF_PDQSR Z0=18-Ohm
MSD_D3RF2_40_PU688   DDR2 MSD_D3R_PDIFF_PDQSR Z0=40-Ohm
MSD_D3RF2_48_PU688   DDR2 MSD_D3R_PDIFF_PDQSR Z0=48-Ohm
MSD_D3RF2_18_PWRDWN   DDR2 MSD_D3R_PDIFF_PDQSR Z0=18-Ohm
MSD_D3RF2_40_PWRDWN   DDR2 MSD_D3R_PDIFF_PDQSR Z0=40-Ohm
MSD_D3RF2_48_PWRDWN   DDR2 MSD_D3R_PDIFF_PDQSR Z0=48-Ohm
MSD_D3RF3_34_OPEN   DDR3 MSD_D3R_PDIFF_PDQSR cell  Z0=34-Ohm
MSD_D3RF3_40_OPEN   DDR3 MSD_D3R_PDIFF_PDQSR cell  Z0=40-Ohm
MSD_D3RF3_48_OPEN   DDR3 MSD_D3R_PDIFF_PDQSR cell  Z0=48-Ohm
MSD_D3RF3_34_PD344   DDR3 MSD_D3R_PDIFF_PDQSR cell  Z0=34-Ohm
MSD_D3RF3_40_PD344   DDR3 MSD_D3R_PDIFF_PDQSR cell  Z0=40-Ohm
MSD_D3RF3_48_PD344   DDR3 MSD_D3R_PDIFF_PDQSR cell  Z0=48-Ohm
MSD_D3RF3_34_PD393   DDR3 MSD_D3R_PDIFF_PDQSR cell  Z0=34-Ohm
MSD_D3RF3_40_PD393   DDR3 MSD_D3R_PDIFF_PDQSR cell  Z0=40-Ohm
MSD_D3RF3_48_PD393   DDR3 MSD_D3R_PDIFF_PDQSR cell  Z0=48-Ohm
MSD_D3RF3_34_PD458   DDR3 MSD_D3R_PDIFF_PDQSR cell  Z0=34-Ohm
MSD_D3RF3_40_PD458   DDR3 MSD_D3R_PDIFF_PDQSR cell  Z0=40-Ohm
MSD_D3RF3_48_PD458   DDR3 MSD_D3R_PDIFF_PDQSR cell  Z0=48-Ohm
MSD_D3RF3_34_PD500   DDR3 MSD_D3R_PDIFF_PDQSR cell  Z0=34-Ohm
MSD_D3RF3_40_PD500   DDR3 MSD_D3R_PDIFF_PDQSR cell  Z0=40-Ohm
MSD_D3RF3_48_PD500   DDR3 MSD_D3R_PDIFF_PDQSR cell  Z0=48-Ohm
MSD_D3RF3_34_PD550   DDR3 MSD_D3R_PDIFF_PDQSR cell  Z0=34-Ohm
MSD_D3RF3_40_PD550   DDR3 MSD_D3R_PDIFF_PDQSR cell  Z0=40-Ohm
MSD_D3RF3_48_PD550   DDR3 MSD_D3R_PDIFF_PDQSR cell  Z0=48-Ohm
MSD_D3RF3_34_PD611   DDR3 MSD_D3R_PDIFF_PDQSR cell  Z0=34-Ohm
MSD_D3RF3_40_PD611   DDR3 MSD_D3R_PDIFF_PDQSR cell  Z0=40-Ohm
MSD_D3RF3_48_PD611   DDR3 MSD_D3R_PDIFF_PDQSR cell  Z0=48-Ohm
MSD_D3RF3_34_PD688   DDR3 MSD_D3R_PDIFF_PDQSR cell  Z0=34-Ohm
MSD_D3RF3_40_PD688   DDR3 MSD_D3R_PDIFF_PDQSR cell  Z0=40-Ohm
MSD_D3RF3_48_PD688   DDR3 MSD_D3R_PDIFF_PDQSR cell  Z0=48-Ohm
MSD_D3RF3_34_PU344   DDR3 MSD_D3R_PDIFF_PDQSR cell  Z0=34-Ohm
MSD_D3RF3_40_PU344   DDR3 MSD_D3R_PDIFF_PDQSR cell  Z0=40-Ohm
MSD_D3RF3_48_PU344   DDR3 MSD_D3R_PDIFF_PDQSR cell  Z0=48-Ohm
MSD_D3RF3_34_PU393   DDR3 MSD_D3R_PDIFF_PDQSR cell  Z0=34-Ohm
MSD_D3RF3_40_PU393   DDR3 MSD_D3R_PDIFF_PDQSR cell  Z0=40-Ohm
MSD_D3RF3_48_PU393   DDR3 MSD_D3R_PDIFF_PDQSR cell  Z0=48-Ohm
MSD_D3RF3_34_PU458   DDR3 MSD_D3R_PDIFF_PDQSR cell  Z0=34-Ohm
MSD_D3RF3_40_PU458   DDR3 MSD_D3R_PDIFF_PDQSR cell  Z0=40-Ohm
MSD_D3RF3_48_PU458   DDR3 MSD_D3R_PDIFF_PDQSR cell  Z0=48-Ohm
MSD_D3RF3_34_PU500   DDR3 MSD_D3R_PDIFF_PDQSR cell  Z0=34-Ohm
MSD_D3RF3_40_PU500   DDR3 MSD_D3R_PDIFF_PDQSR cell  Z0=40-Ohm
MSD_D3RF3_48_PU500   DDR3 MSD_D3R_PDIFF_PDQSR cell  Z0=48-Ohm
MSD_D3RF3_34_PU550   DDR3 MSD_D3R_PDIFF_PDQSR cell  Z0=34-Ohm
MSD_D3RF3_40_PU550   DDR3 MSD_D3R_PDIFF_PDQSR cell  Z0=40-Ohm
MSD_D3RF3_48_PU550   DDR3 MSD_D3R_PDIFF_PDQSR cell  Z0=48-Ohm
MSD_D3RF3_34_PU611   DDR3 MSD_D3R_PDIFF_PDQSR cell  Z0=34-Ohm
MSD_D3RF3_40_PU611   DDR3 MSD_D3R_PDIFF_PDQSR cell  Z0=40-Ohm
MSD_D3RF3_48_PU611   DDR3 MSD_D3R_PDIFF_PDQSR cell  Z0=48-Ohm
MSD_D3RF3_34_PU688   DDR3 MSD_D3R_PDIFF_PDQSR cell  Z0=34-Ohm
MSD_D3RF3_40_PU688   DDR3 MSD_D3R_PDIFF_PDQSR cell  Z0=40-Ohm
MSD_D3RF3_48_PU688   DDR3 MSD_D3R_PDIFF_PDQSR cell  Z0=48-Ohm
MSD_D3RF3_34_PWRDWN   DDR3 MSD_D3R_PDIFF_PDQSR cell  Z0=34-Ohm
MSD_D3RF3_40_PWRDWN   DDR3 MSD_D3R_PDIFF_PDQSR cell  Z0=40-Ohm
MSD_D3RF3_48_PWRDWN   DDR3 MSD_D3R_PDIFF_PDQSR cell  Z0=48-Ohm
MSD_D3RF3L_34_OPEN   DDR3L MSD_D3R_PDIFF_PDQSR cell  Z0=34-Ohm
MSD_D3RF3L_40_OPEN   DDR3L MSD_D3R_PDIFF_PDQSR cell  Z0=40-Ohm
MSD_D3RF3L_48_OPEN   DDR3L MSD_D3R_PDIFF_PDQSR cell  Z0=48-Ohm
MSD_D3RF3L_34_PD344   DDR3L MSD_D3R_PDIFF_PDQSR cell  Z0=34-Ohm
MSD_D3RF3L_40_PD344   DDR3L MSD_D3R_PDIFF_PDQSR cell  Z0=40-Ohm
MSD_D3RF3L_48_PD344   DDR3L MSD_D3R_PDIFF_PDQSR cell  Z0=48-Ohm
MSD_D3RF3L_34_PD393   DDR3L MSD_D3R_PDIFF_PDQSR cell  Z0=34-Ohm
MSD_D3RF3L_40_PD393   DDR3L MSD_D3R_PDIFF_PDQSR cell  Z0=40-Ohm
MSD_D3RF3L_48_PD393   DDR3L MSD_D3R_PDIFF_PDQSR cell  Z0=48-Ohm
MSD_D3RF3L_34_PD458   DDR3L MSD_D3R_PDIFF_PDQSR cell  Z0=34-Ohm
MSD_D3RF3L_40_PD458   DDR3L MSD_D3R_PDIFF_PDQSR cell  Z0=40-Ohm
MSD_D3RF3L_48_PD458   DDR3L MSD_D3R_PDIFF_PDQSR cell  Z0=48-Ohm
MSD_D3RF3L_34_PD500   DDR3L MSD_D3R_PDIFF_PDQSR cell  Z0=34-Ohm
MSD_D3RF3L_40_PD500   DDR3L MSD_D3R_PDIFF_PDQSR cell  Z0=40-Ohm
MSD_D3RF3L_48_PD500   DDR3L MSD_D3R_PDIFF_PDQSR cell  Z0=48-Ohm
MSD_D3RF3L_34_PD550   DDR3L MSD_D3R_PDIFF_PDQSR cell  Z0=34-Ohm
MSD_D3RF3L_40_PD550   DDR3L MSD_D3R_PDIFF_PDQSR cell  Z0=40-Ohm
MSD_D3RF3L_48_PD550   DDR3L MSD_D3R_PDIFF_PDQSR cell  Z0=48-Ohm
MSD_D3RF3L_34_PD611   DDR3L MSD_D3R_PDIFF_PDQSR cell  Z0=34-Ohm
MSD_D3RF3L_40_PD611   DDR3L MSD_D3R_PDIFF_PDQSR cell  Z0=40-Ohm
MSD_D3RF3L_48_PD611   DDR3L MSD_D3R_PDIFF_PDQSR cell  Z0=48-Ohm
MSD_D3RF3L_34_PD688   DDR3L MSD_D3R_PDIFF_PDQSR cell  Z0=34-Ohm
MSD_D3RF3L_40_PD688   DDR3L MSD_D3R_PDIFF_PDQSR cell  Z0=40-Ohm
MSD_D3RF3L_48_PD688   DDR3L MSD_D3R_PDIFF_PDQSR cell  Z0=48-Ohm
MSD_D3RF3L_34_PU344   DDR3L MSD_D3R_PDIFF_PDQSR cell  Z0=34-Ohm
MSD_D3RF3L_40_PU344   DDR3L MSD_D3R_PDIFF_PDQSR cell  Z0=40-Ohm
MSD_D3RF3L_48_PU344   DDR3L MSD_D3R_PDIFF_PDQSR cell  Z0=48-Ohm
MSD_D3RF3L_34_PU393   DDR3L MSD_D3R_PDIFF_PDQSR cell  Z0=34-Ohm
MSD_D3RF3L_40_PU393   DDR3L MSD_D3R_PDIFF_PDQSR cell  Z0=40-Ohm
MSD_D3RF3L_48_PU393   DDR3L MSD_D3R_PDIFF_PDQSR cell  Z0=48-Ohm
MSD_D3RF3L_34_PU458   DDR3L MSD_D3R_PDIFF_PDQSR cell  Z0=34-Ohm
MSD_D3RF3L_40_PU458   DDR3L MSD_D3R_PDIFF_PDQSR cell  Z0=40-Ohm
MSD_D3RF3L_48_PU458   DDR3L MSD_D3R_PDIFF_PDQSR cell  Z0=48-Ohm
MSD_D3RF3L_34_PU500   DDR3L MSD_D3R_PDIFF_PDQSR cell  Z0=34-Ohm
MSD_D3RF3L_40_PU500   DDR3L MSD_D3R_PDIFF_PDQSR cell  Z0=40-Ohm
MSD_D3RF3L_48_PU500   DDR3L MSD_D3R_PDIFF_PDQSR cell  Z0=48-Ohm
MSD_D3RF3L_34_PU550   DDR3L MSD_D3R_PDIFF_PDQSR cell  Z0=34-Ohm
MSD_D3RF3L_40_PU550   DDR3L MSD_D3R_PDIFF_PDQSR cell  Z0=40-Ohm
MSD_D3RF3L_48_PU550   DDR3L MSD_D3R_PDIFF_PDQSR cell  Z0=48-Ohm
MSD_D3RF3L_34_PU611   DDR3L MSD_D3R_PDIFF_PDQSR cell  Z0=34-Ohm
MSD_D3RF3L_40_PU611   DDR3L MSD_D3R_PDIFF_PDQSR cell  Z0=40-Ohm
MSD_D3RF3L_48_PU611   DDR3L MSD_D3R_PDIFF_PDQSR cell  Z0=48-Ohm
MSD_D3RF3L_34_PU688   DDR3L MSD_D3R_PDIFF_PDQSR cell  Z0=34-Ohm
MSD_D3RF3L_40_PU688   DDR3L MSD_D3R_PDIFF_PDQSR cell  Z0=40-Ohm
MSD_D3RF3L_48_PU688   DDR3L MSD_D3R_PDIFF_PDQSR cell  Z0=48-Ohm
MSD_D3RF3L_34_PWRDWN   DDR3L MSD_D3R_PDIFF_PDQSR cell  Z0=34-Ohm
MSD_D3RF3L_40_PWRDWN   DDR3L MSD_D3R_PDIFF_PDQSR cell  Z0=40-Ohm
MSD_D3RF3L_48_PWRDWN   DDR3L MSD_D3R_PDIFF_PDQSR cell  Z0=48-Ohm
MSD_D3RFL2_34_OPEN   LPDDR2 MSD_D3R_PDIFF_PDQSR cell  Z0=34-Ohm
MSD_D3RFL2_40_OPEN   LPDDR2 MSD_D3R_PDIFF_PDQSR cell  Z0=40-Ohm
MSD_D3RFL2_48_OPEN   LPDDR2 MSD_D3R_PDIFF_PDQSR cell  Z0=48-Ohm
MSD_D3RFL2_60_OPEN   LPDDR2 MSD_D3R_PDIFF_PDQSR cell  Z0=60-Ohm
MSD_D3RFL2_80_OPEN   LPDDR2 MSD_D3R_PDIFF_PDQSR cell  Z0=80-Ohm
MSD_D3RFL_48_OPEN   LPDDR MSD_D3R_PDIFF_PDQSR cell  Z0=48-Ohm
MSD_D3RFL2_34_PD344   LPDDR2 MSD_D3R_PDIFF_PDQSR cell  Z0=34-Ohm
MSD_D3RFL2_40_PD344   LPDDR2 MSD_D3R_PDIFF_PDQSR cell  Z0=40-Ohm
MSD_D3RFL2_48_PD344   LPDDR2 MSD_D3R_PDIFF_PDQSR cell  Z0=48-Ohm
MSD_D3RFL2_60_PD344   LPDDR2 MSD_D3R_PDIFF_PDQSR cell  Z0=60-Ohm
MSD_D3RFL2_80_PD344   LPDDR2 MSD_D3R_PDIFF_PDQSR cell  Z0=80-Ohm
MSD_D3RFL_48_PD344   LPDDR MSD_D3R_PDIFF_PDQSR cell  Z0=48-Ohm
MSD_D3RFL2_34_PD393   LPDDR2 MSD_D3R_PDIFF_PDQSR cell  Z0=34-Ohm
MSD_D3RFL2_40_PD393   LPDDR2 MSD_D3R_PDIFF_PDQSR cell  Z0=40-Ohm
MSD_D3RFL2_48_PD393   LPDDR2 MSD_D3R_PDIFF_PDQSR cell  Z0=48-Ohm
MSD_D3RFL2_60_PD393   LPDDR2 MSD_D3R_PDIFF_PDQSR cell  Z0=60-Ohm
MSD_D3RFL2_80_PD393   LPDDR2 MSD_D3R_PDIFF_PDQSR cell  Z0=80-Ohm
MSD_D3RFL_48_PD393   LPDDR MSD_D3R_PDIFF_PDQSR cell  Z0=48-Ohm
MSD_D3RFL2_34_PD458   LPDDR2 MSD_D3R_PDIFF_PDQSR cell  Z0=34-Ohm
MSD_D3RFL2_40_PD458   LPDDR2 MSD_D3R_PDIFF_PDQSR cell  Z0=40-Ohm
MSD_D3RFL2_48_PD458   LPDDR2 MSD_D3R_PDIFF_PDQSR cell  Z0=48-Ohm
MSD_D3RFL2_60_PD458   LPDDR2 MSD_D3R_PDIFF_PDQSR cell  Z0=60-Ohm
MSD_D3RFL2_80_PD458   LPDDR2 MSD_D3R_PDIFF_PDQSR cell  Z0=80-Ohm
MSD_D3RFL_48_PD458   LPDDR MSD_D3R_PDIFF_PDQSR cell  Z0=48-Ohm
MSD_D3RFL2_34_PD500   LPDDR2 MSD_D3R_PDIFF_PDQSR cell  Z0=34-Ohm
MSD_D3RFL2_40_PD500   LPDDR2 MSD_D3R_PDIFF_PDQSR cell  Z0=40-Ohm
MSD_D3RFL2_48_PD500   LPDDR2 MSD_D3R_PDIFF_PDQSR cell  Z0=48-Ohm
MSD_D3RFL2_60_PD500   LPDDR2 MSD_D3R_PDIFF_PDQSR cell  Z0=60-Ohm
MSD_D3RFL2_80_PD500   LPDDR2 MSD_D3R_PDIFF_PDQSR cell  Z0=80-Ohm
MSD_D3RFL_48_PD500   LPDDR MSD_D3R_PDIFF_PDQSR cell  Z0=48-Ohm
MSD_D3RFL2_34_PD550   LPDDR2 MSD_D3R_PDIFF_PDQSR cell  Z0=34-Ohm
MSD_D3RFL2_40_PD550   LPDDR2 MSD_D3R_PDIFF_PDQSR cell  Z0=40-Ohm
MSD_D3RFL2_48_PD550   LPDDR2 MSD_D3R_PDIFF_PDQSR cell  Z0=48-Ohm
MSD_D3RFL2_60_PD550   LPDDR2 MSD_D3R_PDIFF_PDQSR cell  Z0=60-Ohm
MSD_D3RFL2_80_PD550   LPDDR2 MSD_D3R_PDIFF_PDQSR cell  Z0=80-Ohm
MSD_D3RFL_48_PD550   LPDDR MSD_D3R_PDIFF_PDQSR cell  Z0=48-Ohm
MSD_D3RFL2_34_PD611   LPDDR2 MSD_D3R_PDIFF_PDQSR cell  Z0=34-Ohm
MSD_D3RFL2_40_PD611   LPDDR2 MSD_D3R_PDIFF_PDQSR cell  Z0=40-Ohm
MSD_D3RFL2_48_PD611   LPDDR2 MSD_D3R_PDIFF_PDQSR cell  Z0=48-Ohm
MSD_D3RFL2_60_PD611   LPDDR2 MSD_D3R_PDIFF_PDQSR cell  Z0=60-Ohm
MSD_D3RFL2_80_PD611   LPDDR2 MSD_D3R_PDIFF_PDQSR cell  Z0=80-Ohm
MSD_D3RFL_48_PD611   LPDDR MSD_D3R_PDIFF_PDQSR cell  Z0=48-Ohm
MSD_D3RFL2_34_PD688   LPDDR2 MSD_D3R_PDIFF_PDQSR cell  Z0=34-Ohm
MSD_D3RFL2_40_PD688   LPDDR2 MSD_D3R_PDIFF_PDQSR cell  Z0=40-Ohm
MSD_D3RFL2_48_PD688   LPDDR2 MSD_D3R_PDIFF_PDQSR cell  Z0=48-Ohm
MSD_D3RFL2_60_PD688   LPDDR2 MSD_D3R_PDIFF_PDQSR cell  Z0=60-Ohm
MSD_D3RFL2_80_PD688   LPDDR2 MSD_D3R_PDIFF_PDQSR cell  Z0=80-Ohm
MSD_D3RFL_48_PD688   LPDDR MSD_D3R_PDIFF_PDQSR cell  Z0=48-Ohm
MSD_D3RFL2_34_PU344   LPDDR2 MSD_D3R_PDIFF_PDQSR cell  Z0=34-Ohm
MSD_D3RFL2_40_PU344   LPDDR2 MSD_D3R_PDIFF_PDQSR cell  Z0=40-Ohm
MSD_D3RFL2_48_PU344   LPDDR2 MSD_D3R_PDIFF_PDQSR cell  Z0=48-Ohm
MSD_D3RFL2_60_PU344   LPDDR2 MSD_D3R_PDIFF_PDQSR cell  Z0=60-Ohm
MSD_D3RFL2_80_PU344   LPDDR2 MSD_D3R_PDIFF_PDQSR cell  Z0=80-Ohm
MSD_D3RFL_48_PU344   LPDDR MSD_D3R_PDIFF_PDQSR cell  Z0=48-Ohm
MSD_D3RFL2_34_PU393   LPDDR2 MSD_D3R_PDIFF_PDQSR cell  Z0=34-Ohm
MSD_D3RFL2_40_PU393   LPDDR2 MSD_D3R_PDIFF_PDQSR cell  Z0=40-Ohm
MSD_D3RFL2_48_PU393   LPDDR2 MSD_D3R_PDIFF_PDQSR cell  Z0=48-Ohm
MSD_D3RFL2_60_PU393   LPDDR2 MSD_D3R_PDIFF_PDQSR cell  Z0=60-Ohm
MSD_D3RFL2_80_PU393   LPDDR2 MSD_D3R_PDIFF_PDQSR cell  Z0=80-Ohm
MSD_D3RFL_48_PU393   LPDDR MSD_D3R_PDIFF_PDQSR cell  Z0=48-Ohm
MSD_D3RFL2_34_PU458   LPDDR2 MSD_D3R_PDIFF_PDQSR cell  Z0=34-Ohm
MSD_D3RFL2_40_PU458   LPDDR2 MSD_D3R_PDIFF_PDQSR cell  Z0=40-Ohm
MSD_D3RFL2_48_PU458   LPDDR2 MSD_D3R_PDIFF_PDQSR cell  Z0=48-Ohm
MSD_D3RFL2_60_PU458   LPDDR2 MSD_D3R_PDIFF_PDQSR cell  Z0=60-Ohm
MSD_D3RFL2_80_PU458   LPDDR2 MSD_D3R_PDIFF_PDQSR cell  Z0=80-Ohm
MSD_D3RFL_48_PU458   LPDDR MSD_D3R_PDIFF_PDQSR cell  Z0=48-Ohm
MSD_D3RFL2_34_PU500   LPDDR2 MSD_D3R_PDIFF_PDQSR cell  Z0=34-Ohm
MSD_D3RFL2_40_PU500   LPDDR2 MSD_D3R_PDIFF_PDQSR cell  Z0=40-Ohm
MSD_D3RFL2_48_PU500   LPDDR2 MSD_D3R_PDIFF_PDQSR cell  Z0=48-Ohm
MSD_D3RFL2_60_PU500   LPDDR2 MSD_D3R_PDIFF_PDQSR cell  Z0=60-Ohm
MSD_D3RFL2_80_PU500   LPDDR2 MSD_D3R_PDIFF_PDQSR cell  Z0=80-Ohm
MSD_D3RFL_48_PU500   LPDDR MSD_D3R_PDIFF_PDQSR cell  Z0=48-Ohm
MSD_D3RFL2_34_PU550   LPDDR2 MSD_D3R_PDIFF_PDQSR cell  Z0=34-Ohm
MSD_D3RFL2_40_PU550   LPDDR2 MSD_D3R_PDIFF_PDQSR cell  Z0=40-Ohm
MSD_D3RFL2_48_PU550   LPDDR2 MSD_D3R_PDIFF_PDQSR cell  Z0=48-Ohm
MSD_D3RFL2_60_PU550   LPDDR2 MSD_D3R_PDIFF_PDQSR cell  Z0=60-Ohm
MSD_D3RFL2_80_PU550   LPDDR2 MSD_D3R_PDIFF_PDQSR cell  Z0=80-Ohm
MSD_D3RFL_48_PU550   LPDDR MSD_D3R_PDIFF_PDQSR cell  Z0=48-Ohm
MSD_D3RFL2_34_PU611   LPDDR2 MSD_D3R_PDIFF_PDQSR cell  Z0=34-Ohm
MSD_D3RFL2_40_PU611   LPDDR2 MSD_D3R_PDIFF_PDQSR cell  Z0=40-Ohm
MSD_D3RFL2_48_PU611   LPDDR2 MSD_D3R_PDIFF_PDQSR cell  Z0=48-Ohm
MSD_D3RFL2_60_PU611   LPDDR2 MSD_D3R_PDIFF_PDQSR cell  Z0=60-Ohm
MSD_D3RFL2_80_PU611   LPDDR2 MSD_D3R_PDIFF_PDQSR cell  Z0=80-Ohm
MSD_D3RFL_48_PU611   LPDDR MSD_D3R_PDIFF_PDQSR cell  Z0=48-Ohm
MSD_D3RFL2_34_PU688   LPDDR2 MSD_D3R_PDIFF_PDQSR cell  Z0=34-Ohm
MSD_D3RFL2_40_PU688   LPDDR2 MSD_D3R_PDIFF_PDQSR cell  Z0=40-Ohm
MSD_D3RFL2_48_PU688   LPDDR2 MSD_D3R_PDIFF_PDQSR cell  Z0=48-Ohm
MSD_D3RFL2_60_PU688   LPDDR2 MSD_D3R_PDIFF_PDQSR cell  Z0=60-Ohm
MSD_D3RFL2_80_PU688   LPDDR2 MSD_D3R_PDIFF_PDQSR cell  Z0=80-Ohm
MSD_D3RFL_48_PU688   LPDDR MSD_D3R_PDIFF_PDQSR cell  Z0=48-Ohm
MSD_D3RFL2_34_PWRDWN   LPDDR2 MSD_D3R_PDIFF_PDQSR cell  Z0=34-Ohm
MSD_D3RFL2_40_PWRDWN   LPDDR2 MSD_D3R_PDIFF_PDQSR cell  Z0=40-Ohm
MSD_D3RFL2_48_PWRDWN   LPDDR2 MSD_D3R_PDIFF_PDQSR cell  Z0=48-Ohm
MSD_D3RFL2_60_PWRDWN   LPDDR2 MSD_D3R_PDIFF_PDQSR cell  Z0=60-Ohm
MSD_D3RFL2_80_PWRDWN   LPDDR2 MSD_D3R_PDIFF_PDQSR cell  Z0=80-Ohm
MSD_D3RFL_48_PWRDWN   LPDDR MSD_D3R_PDIFF_PDQSR cell  Z0=48-Ohm
MSD_D3RF2_ODT150_OPEN   DDR2 MSD_D3R_PDIFF_PDQSR cell 150-Ohm ODT Receiver
MSD_D3RF2_ODT50_OPEN   DDR2 MSD_D3R_PDIFF_PDQSR cell 50-Ohm ODT Receiver
MSD_D3RF2_ODT75_OPEN   DDR2 MSD_D3R_PDIFF_PDQSR cell 75-Ohm ODT Receiver
MSD_D3RF2_ODTOFF_OPEN   DDR2 MSD_D3R_PDIFF_PDQSR cell ODT off Receiver
MSD_D3RF2_ODT150_PD344   DDR2 MSD_D3R_PDIFF_PDQSR cell 150-Ohm ODT Receiver
MSD_D3RF2_ODT50_PD344   DDR2 MSD_D3R_PDIFF_PDQSR cell 50-Ohm ODT Receiver
MSD_D3RF2_ODT75_PD344   DDR2 MSD_D3R_PDIFF_PDQSR cell 75-Ohm ODT Receiver
MSD_D3RF2_ODTOFF_PD344   DDR2 MSD_D3R_PDIFF_PDQSR cell ODT off Receiver
MSD_D3RF2_ODT150_PD393   DDR2 MSD_D3R_PDIFF_PDQSR cell 150-Ohm ODT Receiver
MSD_D3RF2_ODT50_PD393   DDR2 MSD_D3R_PDIFF_PDQSR cell 50-Ohm ODT Receiver
MSD_D3RF2_ODT75_PD393   DDR2 MSD_D3R_PDIFF_PDQSR cell 75-Ohm ODT Receiver
MSD_D3RF2_ODTOFF_PD393   DDR2 MSD_D3R_PDIFF_PDQSR cell ODT off Receiver
MSD_D3RF2_ODT150_PD458   DDR2 MSD_D3R_PDIFF_PDQSR cell 150-Ohm ODT Receiver
MSD_D3RF2_ODT50_PD458   DDR2 MSD_D3R_PDIFF_PDQSR cell 50-Ohm ODT Receiver
MSD_D3RF2_ODT75_PD458   DDR2 MSD_D3R_PDIFF_PDQSR cell 75-Ohm ODT Receiver
MSD_D3RF2_ODTOFF_PD458   DDR2 MSD_D3R_PDIFF_PDQSR cell ODT off Receiver
MSD_D3RF2_ODT150_PD500   DDR2 MSD_D3R_PDIFF_PDQSR cell 150-Ohm ODT Receiver
MSD_D3RF2_ODT50_PD500   DDR2 MSD_D3R_PDIFF_PDQSR cell 50-Ohm ODT Receiver
MSD_D3RF2_ODT75_PD500   DDR2 MSD_D3R_PDIFF_PDQSR cell 75-Ohm ODT Receiver
MSD_D3RF2_ODTOFF_PD500   DDR2 MSD_D3R_PDIFF_PDQSR cell ODT off Receiver
MSD_D3RF2_ODT150_PD550   DDR2 MSD_D3R_PDIFF_PDQSR cell 150-Ohm ODT Receiver
MSD_D3RF2_ODT50_PD550   DDR2 MSD_D3R_PDIFF_PDQSR cell 50-Ohm ODT Receiver
MSD_D3RF2_ODT75_PD550   DDR2 MSD_D3R_PDIFF_PDQSR cell 75-Ohm ODT Receiver
MSD_D3RF2_ODTOFF_PD550   DDR2 MSD_D3R_PDIFF_PDQSR cell ODT off Receiver
MSD_D3RF2_ODT150_PD611   DDR2 MSD_D3R_PDIFF_PDQSR cell 150-Ohm ODT Receiver
MSD_D3RF2_ODT50_PD611   DDR2 MSD_D3R_PDIFF_PDQSR cell 50-Ohm ODT Receiver
MSD_D3RF2_ODT75_PD611   DDR2 MSD_D3R_PDIFF_PDQSR cell 75-Ohm ODT Receiver
MSD_D3RF2_ODTOFF_PD611   DDR2 MSD_D3R_PDIFF_PDQSR cell ODT off Receiver
MSD_D3RF2_ODT150_PD688   DDR2 MSD_D3R_PDIFF_PDQSR cell 150-Ohm ODT Receiver
MSD_D3RF2_ODT50_PD688   DDR2 MSD_D3R_PDIFF_PDQSR cell 50-Ohm ODT Receiver
MSD_D3RF2_ODT75_PD688   DDR2 MSD_D3R_PDIFF_PDQSR cell 75-Ohm ODT Receiver
MSD_D3RF2_ODTOFF_PD688   DDR2 MSD_D3R_PDIFF_PDQSR cell ODT off Receiver
MSD_D3RF2_ODT150_PU344   DDR2 MSD_D3R_PDIFF_PDQSR cell 150-Ohm ODT Receiver
MSD_D3RF2_ODT50_PU344   DDR2 MSD_D3R_PDIFF_PDQSR cell 50-Ohm ODT Receiver
MSD_D3RF2_ODT75_PU344   DDR2 MSD_D3R_PDIFF_PDQSR cell 75-Ohm ODT Receiver
MSD_D3RF2_ODTOFF_PU344   DDR2 MSD_D3R_PDIFF_PDQSR cell ODT off Receiver
MSD_D3RF2_ODT150_PU393   DDR2 MSD_D3R_PDIFF_PDQSR cell 150-Ohm ODT Receiver
MSD_D3RF2_ODT50_PU393   DDR2 MSD_D3R_PDIFF_PDQSR cell 50-Ohm ODT Receiver
MSD_D3RF2_ODT75_PU393   DDR2 MSD_D3R_PDIFF_PDQSR cell 75-Ohm ODT Receiver
MSD_D3RF2_ODTOFF_PU393   DDR2 MSD_D3R_PDIFF_PDQSR cell ODT off Receiver
MSD_D3RF2_ODT150_PU458   DDR2 MSD_D3R_PDIFF_PDQSR cell 150-Ohm ODT Receiver
MSD_D3RF2_ODT50_PU458   DDR2 MSD_D3R_PDIFF_PDQSR cell 50-Ohm ODT Receiver
MSD_D3RF2_ODT75_PU458   DDR2 MSD_D3R_PDIFF_PDQSR cell 75-Ohm ODT Receiver
MSD_D3RF2_ODTOFF_PU458   DDR2 MSD_D3R_PDIFF_PDQSR cell ODT off Receiver
MSD_D3RF2_ODT150_PU500   DDR2 MSD_D3R_PDIFF_PDQSR cell 150-Ohm ODT Receiver
MSD_D3RF2_ODT50_PU500   DDR2 MSD_D3R_PDIFF_PDQSR cell 50-Ohm ODT Receiver
MSD_D3RF2_ODT75_PU500   DDR2 MSD_D3R_PDIFF_PDQSR cell 75-Ohm ODT Receiver
MSD_D3RF2_ODTOFF_PU500   DDR2 MSD_D3R_PDIFF_PDQSR cell ODT off Receiver
MSD_D3RF2_ODT150_PU550   DDR2 MSD_D3R_PDIFF_PDQSR cell 150-Ohm ODT Receiver
MSD_D3RF2_ODT50_PU550   DDR2 MSD_D3R_PDIFF_PDQSR cell 50-Ohm ODT Receiver
MSD_D3RF2_ODT75_PU550   DDR2 MSD_D3R_PDIFF_PDQSR cell 75-Ohm ODT Receiver
MSD_D3RF2_ODTOFF_PU550   DDR2 MSD_D3R_PDIFF_PDQSR cell ODT off Receiver
MSD_D3RF2_ODT150_PU611   DDR2 MSD_D3R_PDIFF_PDQSR cell 150-Ohm ODT Receiver
MSD_D3RF2_ODT50_PU611   DDR2 MSD_D3R_PDIFF_PDQSR cell 50-Ohm ODT Receiver
MSD_D3RF2_ODT75_PU611   DDR2 MSD_D3R_PDIFF_PDQSR cell 75-Ohm ODT Receiver
MSD_D3RF2_ODTOFF_PU611   DDR2 MSD_D3R_PDIFF_PDQSR cell ODT off Receiver
MSD_D3RF2_ODT150_PU688   DDR2 MSD_D3R_PDIFF_PDQSR cell 150-Ohm ODT Receiver
MSD_D3RF2_ODT50_PU688   DDR2 MSD_D3R_PDIFF_PDQSR cell 50-Ohm ODT Receiver
MSD_D3RF2_ODT75_PU688   DDR2 MSD_D3R_PDIFF_PDQSR cell 75-Ohm ODT Receiver
MSD_D3RF2_ODTOFF_PU688   DDR2 MSD_D3R_PDIFF_PDQSR cell ODT off Receiver
MSD_D3RF2_ODT150_PWRDWN   DDR2 MSD_D3R_PDIFF_PDQSR cell 150-Ohm ODT Receiver
MSD_D3RF2_ODT50_PWRDWN   DDR2 MSD_D3R_PDIFF_PDQSR cell 50-Ohm ODT Receiver
MSD_D3RF2_ODT75_PWRDWN   DDR2 MSD_D3R_PDIFF_PDQSR cell 75-Ohm ODT Receiver
MSD_D3RF2_ODTOFF_PWRDWN   DDR2 MSD_D3R_PDIFF_PDQSR cell ODT off Receiver
MSD_D3RF3_ODT120_OPEN   DDR3 MSD_D3R_PDIFF_PDQSR cell 120-Ohm ODT Receiver
MSD_D3RF3_ODT40_OPEN   DDR3 MSD_D3R_PDIFF_PDQSR cell 40-Ohm ODT Receiver
MSD_D3RF3_ODT60_OPEN   DDR3 MSD_D3R_PDIFF_PDQSR cell 60-Ohm ODT Receiver
MSD_D3RF3_ODTOFF_OPEN   DDR3 MSD_D3R_PDIFF_PDQSR cell ODT off Receiver
MSD_D3RF3_ODT120_PD344   DDR3 MSD_D3R_PDIFF_PDQSR cell 120-Ohm ODT Receiver
MSD_D3RF3_ODT40_PD344   DDR3 MSD_D3R_PDIFF_PDQSR cell 40-Ohm ODT Receiver
MSD_D3RF3_ODT60_PD344   DDR3 MSD_D3R_PDIFF_PDQSR cell 60-Ohm ODT Receiver
MSD_D3RF3_ODTOFF_PD344   DDR3 MSD_D3R_PDIFF_PDQSR cell ODT off Receiver
MSD_D3RF3_ODT120_PD393   DDR3 MSD_D3R_PDIFF_PDQSR cell 120-Ohm ODT Receiver
MSD_D3RF3_ODT40_PD393   DDR3 MSD_D3R_PDIFF_PDQSR cell 40-Ohm ODT Receiver
MSD_D3RF3_ODT60_PD393   DDR3 MSD_D3R_PDIFF_PDQSR cell 60-Ohm ODT Receiver
MSD_D3RF3_ODTOFF_PD393   DDR3 MSD_D3R_PDIFF_PDQSR cell ODT off Receiver
MSD_D3RF3_ODT120_PD458   DDR3 MSD_D3R_PDIFF_PDQSR cell 120-Ohm ODT Receiver
MSD_D3RF3_ODT40_PD458   DDR3 MSD_D3R_PDIFF_PDQSR cell 40-Ohm ODT Receiver
MSD_D3RF3_ODT60_PD458   DDR3 MSD_D3R_PDIFF_PDQSR cell 60-Ohm ODT Receiver
MSD_D3RF3_ODTOFF_PD458   DDR3 MSD_D3R_PDIFF_PDQSR cell ODT off Receiver
MSD_D3RF3_ODT120_PD500   DDR3 MSD_D3R_PDIFF_PDQSR cell 120-Ohm ODT Receiver
MSD_D3RF3_ODT40_PD500   DDR3 MSD_D3R_PDIFF_PDQSR cell 40-Ohm ODT Receiver
MSD_D3RF3_ODT60_PD500   DDR3 MSD_D3R_PDIFF_PDQSR cell 60-Ohm ODT Receiver
MSD_D3RF3_ODTOFF_PD500   DDR3 MSD_D3R_PDIFF_PDQSR cell ODT off Receiver
MSD_D3RF3_ODT120_PD550   DDR3 MSD_D3R_PDIFF_PDQSR cell 120-Ohm ODT Receiver
MSD_D3RF3_ODT40_PD550   DDR3 MSD_D3R_PDIFF_PDQSR cell 40-Ohm ODT Receiver
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| Models and submodels in the file (581): io8_ft_et_fs_1v2 (I/O), io8_ft_et_hs_1v2 (I/O), io8_ft_et_hslv_fs_1v2 (I/O), io8_ft_et_hslv_hs_1v2 (I/O), io8_ft_et_hslv_ls_1v2 (I/O), io8_ft_et_hslv_ms_1v2 (I/O), io8_ft_et_ls_1v2 (I/O), io8_ft_et_ms_1v2 (I/O), io8_ft_fs_1v2 (I/O), io8_ft_hs_1v2 (I/O), io8_ft_hslv_fs_1v2 (I/O), io8_ft_hslv_hs_1v2 (I/O), io8_ft_hslv_ls_1v2 (I/O), io8_ft_hslv_ms_1v2 (I/O), io8_ft_i2c_1v2 (I/O_open_drain), io8_ft_i2c_hslv_1v2 (I/O_open_drain), io8_ft_ls_1v2 (I/O), io8_ft_ms_1v2 (I/O), isudqf_ft_1v2 (Input), io8_ft_et_fs_1v8 (I/O), io8_ft_et_hs_1v8 (I/O), io8_ft_et_hslv_fs_1v8 (I/O), io8_ft_et_hslv_hs_1v8 (I/O), io8_ft_et_hslv_ls_1v8 (I/O), io8_ft_et_hslv_ms_1v8 (I/O), io8_ft_et_ls_1v8 (I/O), io8_ft_et_ms_1v8 (I/O), io8_ft_fs_1v8 (I/O), io8_ft_hs_1v8 (I/O), io8_ft_hslv_fs_1v8 (I/O), io8_ft_hslv_hs_1v8 (I/O), io8_ft_hslv_ls_1v8 (I/O), io8_ft_hslv_ms_1v8 (I/O), io8_ft_i2c_1v8 (I/O_open_drain), io8_ft_i2c_hslv_1v8 (I/O_open_drain), io8_ft_ls_1v8 (I/O), io8_ft_ms_1v8 (I/O), isudqf_ft_1v8 (Input), io8_ft_et_hslv_fs_2v5 (I/O), io8_ft_et_hslv_hs_2v5 (I/O), io8_ft_et_hslv_ls_2v5 (I/O), io8_ft_et_hslv_ms_2v5 (I/O), io8_ft_hslv_fs_2v5 (I/O), io8_ft_hslv_hs_2v5 (I/O), io8_ft_hslv_ls_2v5 (I/O), io8_ft_hslv_ms_2v5 (I/O), io8_ft_i2c_hslv_2v5 (I/O_open_drain), io8_ft_et_fs_3v3 (I/O), io8_ft_et_hs_3v3 (I/O), io8_ft_et_ls_3v3 (I/O), io8_ft_et_ms_3v3 (I/O), io8_ft_fs_3v3 (I/O), io8_ft_hs_3v3 (I/O), io8_ft_i2c_3v3 (I/O_open_drain), io8_ft_ls_3v3 (I/O), io8_ft_ms_3v3 (I/O), io8usb_ft_hs_3v3 (I/O), io8usb_ft_ls_3v3 (I/O), isudqf_ft_3v3 (Input), MSD_D3RF2_18 (I/O), MSD_D3RF2_40 (I/O), MSD_D3RF2_48 (I/O), MSD_D3RF2_ODT150 (Input), MSD_D3RF2_ODT50 (Input), MSD_D3RF2_ODT75 (Input), MSD_D3RF2_ODTOFF (Input), MSD_D3RF3_34 (I/O), MSD_D3RF3_40 (I/O), MSD_D3RF3_48 (I/O), MSD_D3RF3L_34 (I/O), MSD_D3RF3L_40 (I/O), MSD_D3RF3L_48 (I/O), MSD_D3RF3L_ODT120 (Input), MSD_D3RF3L_ODT40 (Input), MSD_D3RF3L_ODT60 (Input), MSD_D3RF3L_ODTOFF (Input), MSD_D3RF3_ODT120 (Input), MSD_D3RF3_ODT40 (Input), MSD_D3RF3_ODT60 (Input), MSD_D3RF3_ODTOFF (Input)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
